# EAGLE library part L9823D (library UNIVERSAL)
L9823D - Automotive low side swwitch.
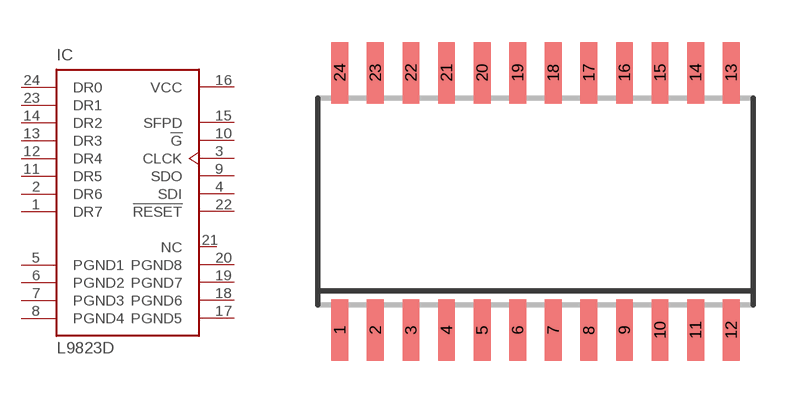
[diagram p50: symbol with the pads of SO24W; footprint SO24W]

Designator prefix IC

## L9823D (IC: l9823d)  [SO24W]
1  DR7
2  DR6
3  CLCK  in
4  SDI  in
5  PGND1  pwr
6  PGND2  pwr
7  PGND3  pwr
8  PGND4  pwr
9  SDO  out
10  !G  in
11  DR5
12  DR4
13  DR3
14  DR2
15  SFPD  out
16  VCC  pwr
17  PGND5  pwr
18  PGND6  pwr
19  PGND7  pwr
20  PGND8  pwr
21  NC  nc
22  !RESET  in
23  DR1
24  DR0

## Footprint SO24W (pad centres in mm)
smd 0.6 x 2.2: 1 0.635,-0.79; 2 1.905,-0.79; 3 3.175,-0.79; 4 4.445,-0.79; 5 5.715,-0.79; 6 6.985,-0.79; 7 8.255,-0.79; 8 9.525,-0.79; 9 10.795,-0.79; 10 12.065,-0.79; 11 13.335,-0.79; 12 14.605,-0.79; 13 14.605,8.41; 14 13.335,8.41; 15 12.065,8.41; 16 10.795,8.41; 17 9.525,8.41; 18 8.255,8.41; 19 6.985,8.41; 20 5.715,8.41; 21 4.445,8.41; 22 3.175,8.41; 23 1.905,8.41; 24 0.635,8.41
